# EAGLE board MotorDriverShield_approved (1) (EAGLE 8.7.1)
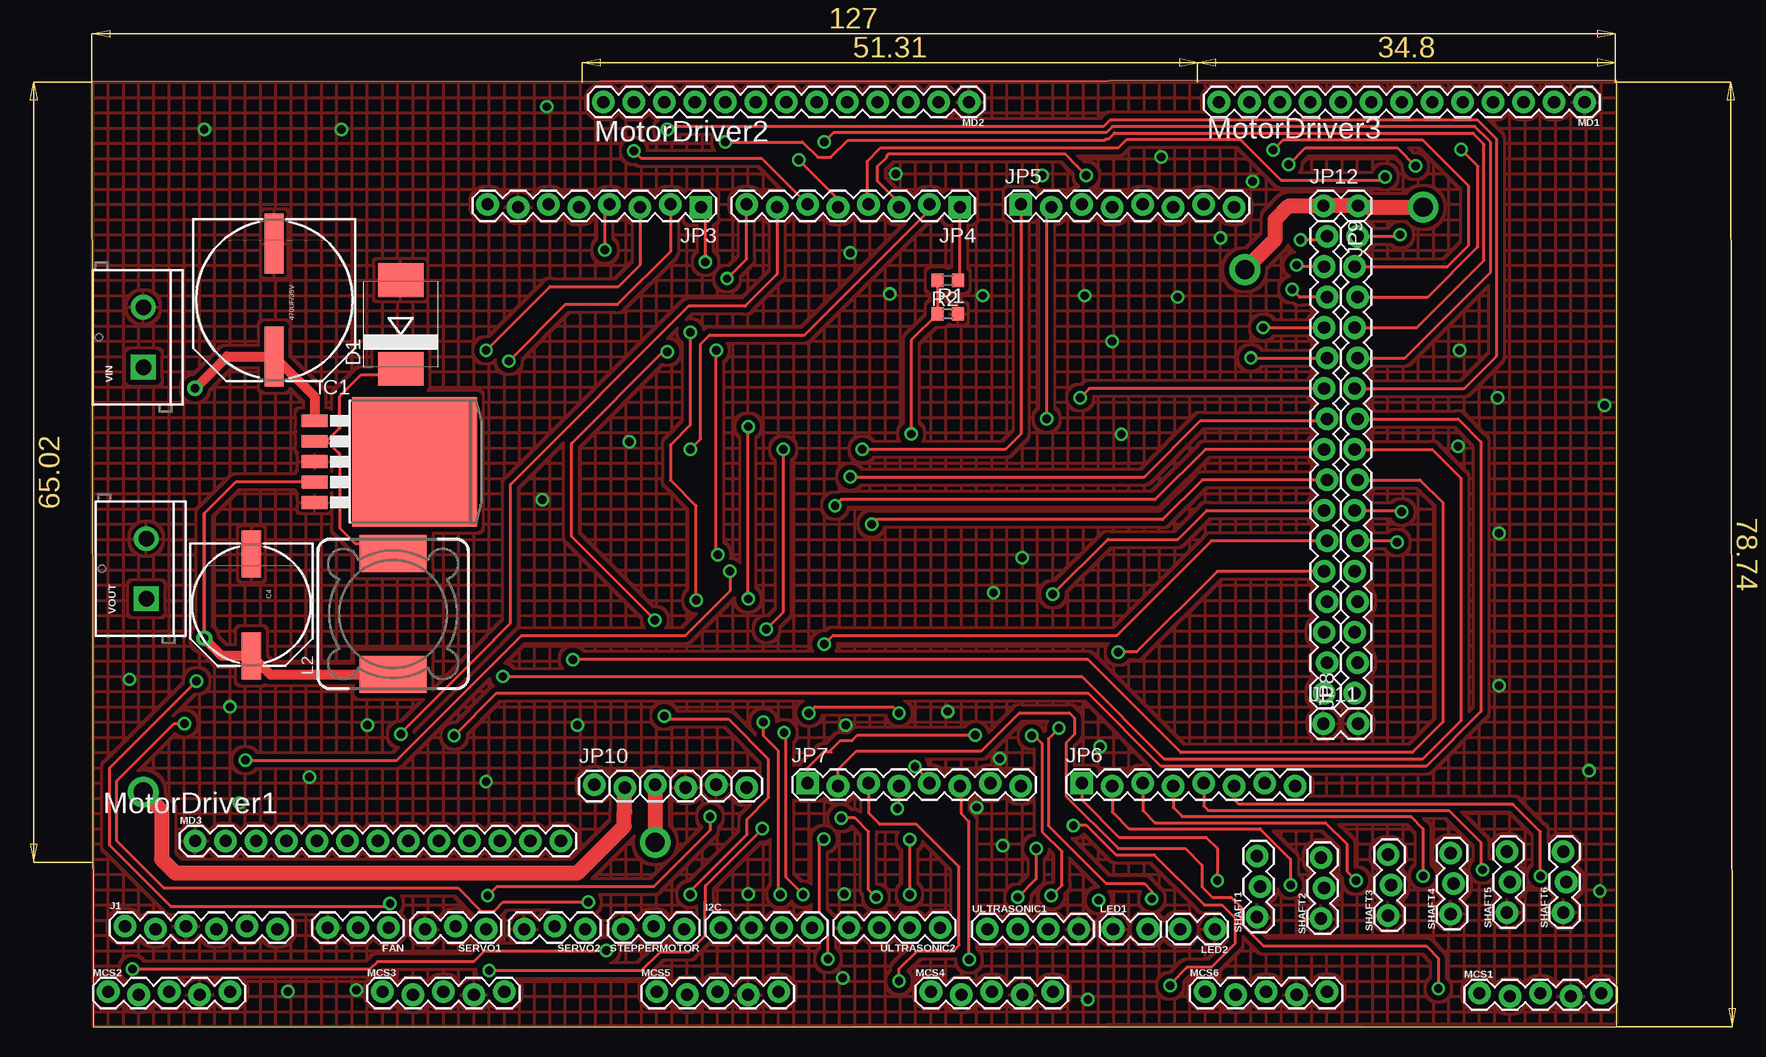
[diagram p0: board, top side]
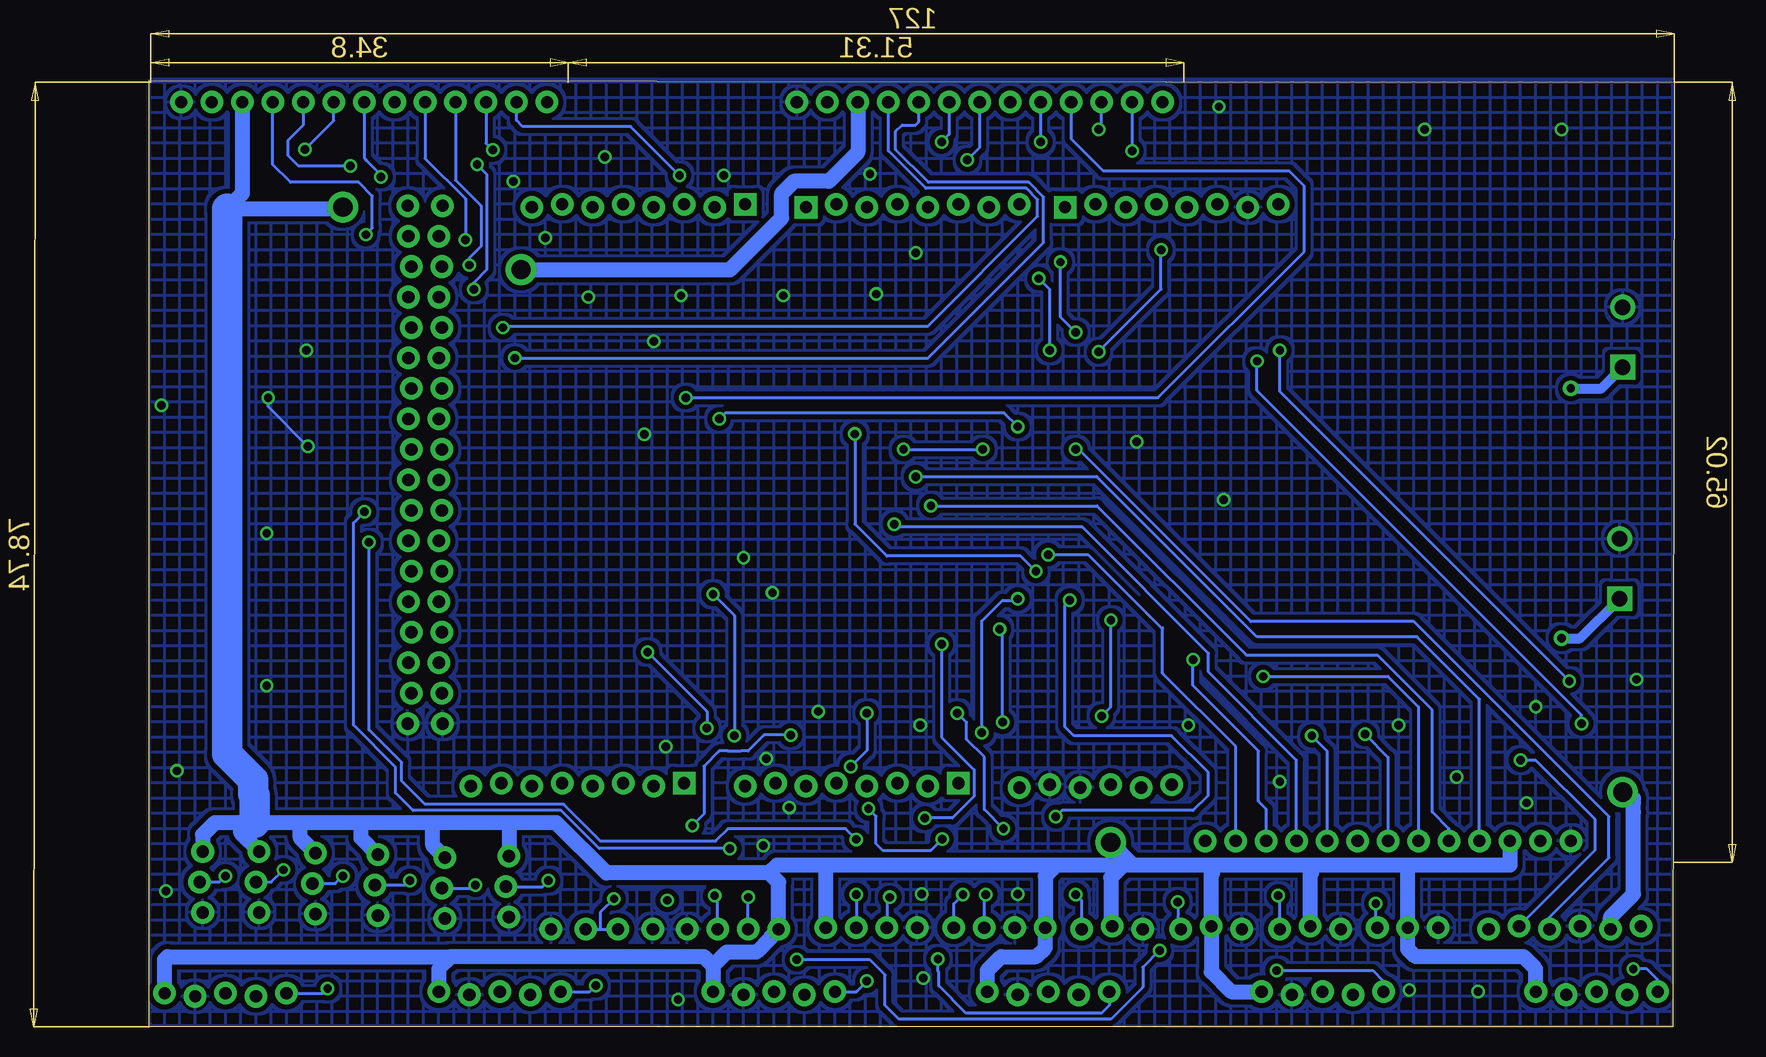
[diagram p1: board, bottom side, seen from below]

Size 142.2 x 83.1 mm. Coordinates in mm from the lower left corner, seen from the top.
Outline: 132.25,78.87 5.13,78.74 5.25,0 132.25,0 132.25,78.87
Copper layers (1*16): Top 0.035mm / dielectric 1.5mm / Bottom 0.035mm
Design rules "Voltera_DRC": minimum track width 10mil, minimum drill 0.6mm, track to track 10mil, track to pad 10mil, pad to pad 0.6mm, via to via 0.6mm, smd to smd 0mil, copper to edge 0mil, drill to drill 0.8mm, minimum pad ring 0.2mm, minimum via ring 0.2mm, stop-mask expansion 4mil, vias tented up to drill 0mil, thermal gap 10mil

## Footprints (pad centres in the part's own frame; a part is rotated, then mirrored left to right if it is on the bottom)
CPOL_PANASONIC_H13 = smd 5 x 1.6: + 4.7,0; - -4.7,0
CPOL_PANASONIC_G = smd 3.9 x 1.6: + 4.25,0; - -4.25,0
SMC = smd 2.8 x 3.8: A 3.7,0; C -3.7,0
1X03 = drill 1.016 pad 1.88: 1 0,0; 2 2.54,0; 3 5.08,0
1X04 = drill 1.016 pad 1.88: 1 0,0; 2 2.54,0; 3 5.08,0; 4 7.62,0
TO263-5 = smd 1.067 x 2.159: 1 -3.404,-5.791; 2 -1.702,-5.791; 3 0,-5.791; 4 1.702,-5.791; 5 3.404,-5.791 | smd 10.8 x 10.41: 6 0,2.54
1X06_LOCK = drill 1.016 pad 1.88: 1 0,0; 2 2.54,-0.254; 3 5.08,0; 4 7.62,-0.254; 5 10.16,0; 6 12.7,-0.254
1X08_LOCK = drill 1.016 pad 1.88 square: 1 0,0.127 | drill 1.016 pad 1.88: 2 2.54,-0.127; 3 5.08,0.127; 4 7.62,-0.127; 5 10.16,0.127; 6 12.7,-0.127; 7 15.24,0.127; 8 17.78,-0.127
1X16_LOCK = drill 1.016 pad 1.88: 1 0,0.127; 2 2.54,-0.127; 3 5.08,0.127; 4 7.62,-0.127; 5 10.16,0.127; 6 12.7,-0.127; 7 15.24,0.127; 8 17.78,-0.127; 9 20.32,0.127; 10 22.86,-0.127; 11 25.4,0.127; 12 27.94,-0.127; 13 30.48,0.127; 14 33.02,-0.127; 15 35.56,0.127; 16 38.1,-0.127
1X02_LOCK = drill 1.016 pad 1.88: 1 -0.178,0; 2 2.718,0
SRR1210 = smd 5.6 x 3.1: 1 0,5.05; 2 0,-5.05
1X05_LOCK = drill 1.016 pad 1.88: 1 0,0.127; 2 2.54,-0.127; 3 5.08,0.127; 4 7.62,-0.127; 5 10.16,0.127
1X13 = drill 1.016 pad 1.88: 1 0,0; 2 2.54,0; 3 5.08,0; 4 7.62,0; 5 10.16,0; 6 12.7,0; 7 15.24,0; 8 17.78,0; 9 20.32,0; 10 22.86,0; 11 25.4,0; 12 27.94,0; 13 30.48,0
R0603 = smd 1 x 1.1: 1 -0.85,0; 2 0.85,0
1X03_LOCK = drill 1.016 pad 1.88: 1 0,0.127; 2 2.54,-0.127; 3 5.08,0.127
SCREWTERMINAL-5MM-2 = drill 1.3 pad 2.032 square: 1 0,0 | drill 1.3 pad 2.032: 2 5,0

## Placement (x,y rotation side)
470UF/35V  [CPOL_PANASONIC_H13]  20.37,60.58 270 top
C4  220uf/25v  [CPOL_PANASONIC_G]  18.46,35.18 270 top
D1  [SMC]  30.91,58.55 90 top
FAN  [1X03]  29.89,8.26 180 top
I2C  [1X04]  57.58,8.26 0 top
IC1  LM2596S  [TO263-5]  29.51,47.12 270 top
J1  [1X06_LOCK]  7.92,8.38 0 top
JP3  [1X08_LOCK]  55.93,68.45 180 top
JP4  [1X08_LOCK]  77.52,68.45 180 top
JP5  [1X08_LOCK]  82.6,68.45 0 top
JP6  [1X08_LOCK]  87.68,20.19 0 top
JP7  [1X08_LOCK]  64.82,20.19 0 top
JP8  M16LOCK  [1X16_LOCK]  110.54,27.81 90 top
JP9  M16LOCK  [1X16_LOCK]  108,65.91 270 top
JP10  [1X06_LOCK]  47.04,20.19 0 top
JP11  [1X02_LOCK]  108,25.27 0 top
JP12  [1X02_LOCK]  108,68.45 0 top
L2  SRR1210  [SRR1210]  30.27,34.42 0 top
LED1  [1X02_LOCK]  90.47,8.13 0 top
LED2  [1X02_LOCK]  98.6,8.13 180 top
MCS1  [1X05_LOCK]  120.82,2.67 0 top
MCS2  [1X05_LOCK]  6.52,2.79 0 top
MCS3  [1X05_LOCK]  29.38,2.79 0 top
MCS4  [1X05_LOCK]  75.1,2.79 0 top
MCS5  [1X05_LOCK]  52.24,2.79 0 top
MCS6  [1X05_LOCK]  97.96,2.79 0 top
MD1  [1X13]  129.59,77.09 180 top
MD2  [1X13]  78.28,77.09 180 top
MD3  [1X13]  13.76,15.49 0 top
R1  1k  [R0603]  76.5,59.44 0 top
R2  2k  [R0603]  76.5,62.23 180 top
SERVO1  [1X03_LOCK]  38.02,8.26 180 top
SERVO2  [1X03_LOCK]  46.27,8.26 180 top
SHAFT1  [1X03_LOCK]  102.41,9.14 90 top
SHAFT2  [1X03_LOCK]  107.74,9.02 90 top
SHAFT3  [1X03_LOCK]  113.33,9.27 90 top
SHAFT4  [1X03_LOCK]  118.54,9.4 90 top
SHAFT5  [1X03_LOCK]  123.24,9.53 90 top
SHAFT6  [1X03_LOCK]  127.94,9.53 90 top
STEPPERMOTOR  [1X03_LOCK]  54.53,8.26 180 top
ULTRASONIC1  [1X04]  79.8,8.13 0 top
ULTRASONIC2  [1X04]  75.86,8.26 180 top
VIN  [SCREWTERMINAL-5MM-2]  9.44,54.99 90 top
VOUT  [SCREWTERMINAL-5MM-2]  9.7,35.69 90 top

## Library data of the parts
470UF/35V C4 = ELL-i-Passive
D1 = diode
FAN J1 LED1 LED2 MCS1-MCS6 MD1-MD3 SERVO1 SERVO2 SHAFT1-SHAFT6 STEPPERMOTOR = SparkFun-Connectors
I2C ULTRASONIC1 ULTRASONIC2 = SparkFun-Connectors; PROD_ID: CONN-09696
IC1 = national-semiconductor; MF: NATIONAL SEMICONDUCTOR; MPN: LM2596S-ADJ/NOPB; OC_FARNELL: 9494367; OC_NEWARK: 41K3842
JP3-JP12 = SparkFun
L2 = inductor-bourns
R1 R2 = audio amplifier example
VIN VOUT = SparkFun-Connectors; SF_SKU: PRT-08432

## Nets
3.3: J1.2 JP10.2
5V: FAN.2 I2C.1 JP10.3 JP12.1 JP12.2 MCS1.5 MCS2.5 MCS3.5 MCS4.5 MCS5.5 MCS6.5 MD1.3 MD2.3 MD3.3 SERVO1.2 SERVO2.2 SHAFT1.3 SHAFT2.3 SHAFT3.3 SHAFT4.3 SHAFT5.3 SHAFT6.3 STEPPERMOTOR.2 ULTRASONIC1.1 ULTRASONIC2.1
A0: JP7.1 MCS6.1
A1: JP7.2 MCS1.1
A2: JP7.3 MCS4.1
A3: JP7.4 MCS5.1
A4: JP7.5 MCS3.1
A5: JP7.6 MCS2.1
A6: JP7.7
A7: JP7.8
A8: JP6.1 SHAFT1.2
A9: JP6.2 SHAFT2.2
A10: JP6.3 SHAFT3.2
A11: JP6.4 SHAFT4.2
A12: JP6.5 SHAFT5.2
A13: JP6.6 SHAFT6.2
A14: JP6.7
A15: JP6.8
AREF: JP3.8
D2: JP4.3 MD1.12
D3: JP4.4 MD1.7
D4: JP4.5 MD2.7
D5: JP4.6 MD2.12
D6: JP4.7 MD3.7
D7: JP4.8 MD3.12
D8: JP3.1 SERVO1.1
D9: JP3.2 SERVO2.1
D10: FAN.1 JP3.3
D11: JP3.4 STEPPERMOTOR.1
D12: JP3.5
D13: JP3.6
D14: JP5.8
D15: JP5.7
D16: JP5.6
D17: JP5.5
D18: JP5.4
D19: JP5.3
D22: JP9.1 MD1.9
D23: JP8.16 MD1.4
D24: JP9.2 MD1.10
D25: JP8.15 MD1.11
D26: JP9.3 MD1.5
D27: JP8.14 MD1.6
D28: JP9.4 MD2.4
D29: JP8.13 MD2.9
D30: JP9.5 MD2.5
D31: JP8.12 MD2.6
D32: JP9.6 MD2.10
D33: JP8.11 MD2.11
D34: JP9.7 MD3.4
D35: JP8.10 MD3.9
D36: JP9.8 MD3.5
D37: JP8.9 MD3.6
D38: JP9.9 MD3.10
D39: JP8.8 MD3.11
D40: JP9.10 ULTRASONIC1.3
D41: JP8.7 ULTRASONIC1.2
D42: JP9.11 ULTRASONIC2.3
D43: JP8.6 ULTRASONIC2.2
D44: JP9.12 LED1.2 LED2.2
D45: JP8.5
D46: JP9.13
D47: JP8.4
D48: JP9.14
D49: JP8.3
D50: JP9.15
D51: JP8.2
D52: JP9.16
D53: JP8.1
EN: J1.1
GND: 470UF/35V.- C4.- D1.A FAN.3 I2C.2 IC1.3 IC1.5 J1.3 JP3.7 JP10.4 JP10.5 JP11.1 JP11.2 LED1.1 LED2.1 MCS1.4 MCS2.4 MCS3.4 MCS4.4 MCS5.4 MCS6.4 MD1.1 MD2.1 MD3.1 R1.2 SERVO1.3 SERVO2.3 SHAFT1.1 SHAFT2.1 SHAFT3.1 SHAFT4.1 SHAFT5.1 SHAFT6.1 STEPPERMOTOR.3 ULTRASONIC1.4 ULTRASONIC2.4 VIN.2 VOUT.2
OUT: D1.C IC1.2 L2.1
PVIN: 470UF/35V.+ IC1.1 VIN.1
PVOUT: C4.+ IC1.4 L2.2 VOUT.1
RES: JP10.1
RX: JP4.1 R2.1
RX0: J1.5 R1.1 R2.2
SCL: I2C.3 JP5.1
SDA: I2C.4 JP5.2
STATE: J1.6
TX: J1.4 JP4.2
VIN: JP10.6

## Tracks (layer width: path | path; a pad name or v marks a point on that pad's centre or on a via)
3.3  (via drill 1.6)
  Top 1.27: JP10.2 49.58,17.95 49.53,17.91 49.53,16.72 45.64,12.83 12.11,12.83 10.97,13.97 10.97,18.03 v9.44,19.56
  Bottom 1.27: J1.2 10.46,9.14 8.55,11.05 8.55,17.91 8.55,18.67 | 8.55,18.67 8.55,19.05 | 8.55,18.67 v9.44,19.56
5V  (via drill 1.6)
  Top 1.27: v101.27,63.12 103.81,65.66 103.81,67.31 104.95,68.45 JP12.1 JP12.2 110.84,68.33 v116.12,68.33 | JP10.3 v52.12,15.37
  Bottom 1.27: 102.03,17.02 98.34,17.02 94.15,12.83 80.58,12.83 | 102.03,17.02 108.63,17.02 | 108.63,17.02 114.6,17.02 | 114.6,17.02 119.68,17.02 | 119.68,17.02 123.49,17.02 124.63,17.02 | SHAFT2.3 108.63,15.11 108.63,17.02 | SHAFT3.3 114.6,15.75 114.6,17.02 | SHAFT4.3 119.68,15.75 119.68,17.02 | SHAFT5.3 124.63,16.13 124.63,17.02 | MD1.3 124.51,69.47 125.78,68.2 116.25,68.2 v116.12,68.33 | SERVO1.2 35.48,12.7 | 35.48,12.7 35.35,12.83 | 43.73,12.7 SERVO2.2 43.73,4.57 42.08,2.92 MCS3.5 | 43.73,12.7 43.61,12.83 | 102.03,17.02 102.28,16.76 SHAFT1.3 | 124.63,17.02 126.79,17.02 127.81,16 SHAFT6.3 | MD3.3 18.84,13.46 27.48,13.46 | MD2.3 73.2,72.9 75.61,70.48 78.53,70.48 79.55,69.47 79.55,67.44 83.87,63.12 v101.27,63.12 | 27.48,13.46 35.35,13.46 | 35.35,13.46 43.99,13.46 | 27.48,13.46 27.35,13.34 FAN.2 27.35,6.48 26.72,5.84 17.7,5.84 16.68,4.83 MCS2.5 16.68,3.43 | 35.48,12.7 35.48,13.34 35.35,13.46 | 43.73,12.7 43.73,13.21 43.99,13.46 | 50.21,13.46 v52.12,15.37 | 43.99,13.46 50.21,13.46 | 50.21,13.46 51.1,13.46 | 51.1,13.46 52.12,12.45 52.12,8.51 STEPPERMOTOR.2 | 51.1,13.46 56.69,13.46 | 56.69,13.46 57.58,12.57 I2C.1 57.58,6.6 58.34,5.84 61.26,5.84 62.4,4.7 MCS5.5 | 56.69,13.46 75.74,13.46 | 75.74,13.46 79.95,13.46 80.58,12.83 | 75.74,13.46 75.86,13.34 ULTRASONIC2.1 | 80.58,12.83 79.8,12.05 ULTRASONIC1.1 80.51,7.42 80.51,7.37 81.66,6.22 84.12,6.22 85.26,5.08 | 85.26,5.08 MCS4.5 | 85.26,5.08 86.03,5.84 107.11,5.84 | MCS6.5 108.12,4.83 107.11,5.84 | MCS1.5 130.98,5.59 130.73,5.84 107.11,5.84
  Bottom 2.54: 123.49,17.02 123.49,19.3 123.62,19.43 123.62,20.57 125.78,22.73 125.78,68.2
A0  (via drill 0.7)
  Top 0.254: JP7.1 64.82,21.59 66.13,22.91 66.59,22.91 | v86.98,16.78 88.08,16.78 90.51,14.35 93.69,14.35 97.88,10.16 99.36,10.16 100.45,9.07 100.45,6.93 98.47,4.95 96.44,4.95 95.04,3.56 v95.04,3.43 | 66.8,22.91 66.59,22.91 | 66.59,22.91 67.55,23.86 68.52,23.86 68.98,24.32 v78.8,24.32
  Bottom 0.254: v78.8,24.32 81.01,24.32 82.34,22.99 82.94,22.99 82.95,22.97 84.02,22.97 84.03,22.99 84.75,22.99 86.03,21.72 86.03,17.73 v86.98,16.78 | MCS6.1 95.55,2.92 v95.04,3.43
A1  (via drill 0.7)
  Top 0.254: JP7.2 67.36,21.46 68.88,22.99 79.29,22.99 82.49,26.18 86.64,26.18 87.06,25.76 87.06,24.36 86.36,23.66 86.36,19.22 90.72,14.86 96.31,14.86 97.69,13.48 97.69,11.66 98.56,10.79 100.12,10.79 100.96,9.96 100.96,8.6 102.83,6.73 116.38,6.73 117.39,5.71 v117.39,3.17
  Bottom 0.254: MCS1.1 117.78,2.79 v117.39,3.17
A2  (via drill 0.7)
  Top 0.254: JP7.3 69.9,17.82 70.81,16.91 73.86,16.91 77.45,13.31 77.45,6.79 77.01,6.35 73.96,6.35 72.44,4.83 v72.44,3.81
  Bottom 0.254: MCS4.1 73.33,2.92 v72.44,3.81
A3  (via drill 0.7)
  Top 0.254: v66.52,5.64 66.52,8.8 65.83,9.49 65.83,15.29 v66.18,15.64 | v72.31,18.2 72.44,18.32 JP7.4
  Bottom 0.254: v72.31,18.2 71.67,17.56 71.67,15.24 71.15,14.71 67.1,14.71 v66.18,15.64 | MCS5.1 52.24,1.78 52.88,1.14 64.18,1.14 66.45,3.41 66.45,4.6 66.52,4.67 v66.52,5.64
A4  (via drill 0.7)
  Top 0.254: v61.06,16.51 56.31,11.76 56.31,11.58 56.32,11.56 56.32,10.5 56.26,10.43 56.26,7.71 56.31,7.66 56.31,7.62 54.91,6.22 52.52,6.22 51,4.7 v38.27,4.7 | v64.93,26.16 65.43,26.67 71.93,26.67 v72.44,26.16 | v73.77,21.7 74.98,20.5 JP7.5
  Bottom 0.254: v61.06,16.51 62.66,18.11 62.66,22.5 64.14,23.98 64.14,25.38 v64.93,26.16 | v72.44,26.16 72.44,23.04 v73.77,21.7 | MCS3.1 29.38,3.81 30.27,4.7 v38.27,4.7
A5  (via drill 0.7)
  Top 0.254: v78.28,5.59 78.28,17.1 77.63,17.75 77.63,19.96 JP7.6 | v8.55,4.83 28.37,4.83 28.96,5.42 36.96,5.42 37.89,6.35 47.16,6.35 47.18,6.37 v48.05,6.37
  Bottom 0.254: v78.28,5.59 72.18,5.59 70.91,4.32 70.91,1.78 69.77,0.64 52.12,0.64 49.45,3.3 49.45,4.97 v48.05,6.37 | MCS2.1 6.52,3.94 7.41,4.83 v8.55,4.83
A8  (via drill 0.7)
  Top 0.254: JP6.1 87.68,18.92 90.79,15.81 98.03,15.81 98.98,14.86 v98.98,12.19
  Bottom 0.254: SHAFT1.2 99.49,11.68 v98.98,12.19
A9  (via drill 0.7)
  Top 0.254: JP6.2 90.22,17.91 91.61,16.51 102.53,16.51 105.08,13.97 v105.08,11.81
  Bottom 0.254: SHAFT2.2 105.33,11.56 v105.08,11.81
A10  (via drill 0.7)
  Top 0.254: JP6.3 92.76,18.03 93.77,17.02 108,17.02 109.77,15.24 109.77,12.95 v110.54,12.19
  Bottom 0.254: v110.54,12.19 110.92,11.81 SHAFT3.2
A11  (via drill 0.7)
  Top 0.254: JP6.4 95.3,18.29 96.06,17.53 115.11,17.53 116.12,16.51 v116.12,12.57
  Bottom 0.254: SHAFT4.2 116.76,11.94 v116.12,12.57
A12  (via drill 0.7)
  Top 0.254: JP6.5 97.84,18.41 98.22,18.03 118.28,18.03 120.95,15.37 120.95,13.21 v121.08,13.08
  Bottom 0.254: SHAFT5.2 122.09,12.06 v121.08,13.08
A13  (via drill 0.7)
  Top 0.254: v125.9,12.57 125.9,16.26 123.62,18.54 100.76,18.54 100.38,18.92 JP6.6
  Bottom 0.254: SHAFT6.2 126.41,12.06 v125.9,12.57
D2  (via drill 0.7)
  Top 0.254: 87.28,71.75 87.29,71.75 | 87.29,71.75 v88.06,70.98 | 87.29,71.75 87.29,71.76 86.28,72.77 75.86,72.77 75.48,72.77 71.55,72.77 71.42,72.64 71.42,72.52 70.66,71.75 70.66,70.48 72.44,68.71 JP4.3
  Bottom 0.254: MD1.12 101.65,75.56 101.14,75.06 92.14,75.06 v88.06,70.98
D3  (via drill 0.7)
  Top 0.254: JP4.4 69.77,68.71 69.77,72.14 70.91,73.28 90.72,73.28 91.44,74 100.87,74 104.27,70.59 112.68,70.59 v112.95,70.87
  Bottom 0.254: 112.95,71.03 112.95,70.99 | 112.95,70.99 v112.95,70.87 | MD1.7 114.35,72.43 114.2,72.29 114.2,72.25 112.95,70.99
D4  (via drill 0.7)
  Top 0.254: v64.07,72.28 67.36,68.99 JP4.5
  Bottom 0.254: MD2.7 63.04,73.31 v64.07,72.28
D5  (via drill 0.7)
  Top 0.254: JP4.6 61.01,72.39 50.97,72.39 v50.34,73.03
  Bottom 0.254: MD2.12 v50.34,73.03
D6  (via drill 0.7)
  Top 0.254: JP4.7 62.28,62.74 59.61,60.07 54.91,60.07 40.05,45.21 40.05,33.66 38.65,32.26 38.65,32.23 30.91,24.48 v30.91,24.38
  Bottom 0.254: v30.91,24.38 29,22.48 MD3.7
D7  (via drill 0.7)
  Top 0.254: v57.32,39.37 57.2,39.5 v57.2,56.39 | v58.11,62.38 59.74,64.01 JP4.8
  Bottom 0.254: v57.2,56.39 57.2,61.47 v58.11,62.38 | 47.8,33.15 47.8,29.46 41.7,23.37 MD3.12 | 47.8,33.15 47.8,33.27 | 47.8,33.15 54.02,39.37 v57.32,39.37
D8  (via drill 0.7)
  Top 0.254: v38.15,10.92 38.91,11.68 51.99,11.68 56.69,16.38 v56.69,17.53 | v55.53,35.56 55.53,43.43 53.39,45.58 53.39,48.51 55.04,50.16 v55.04,57.91 | v56.31,63.75 56.31,67.94 JP3.1
  Bottom 0.254: SERVO1.1 38.02,10.79 v38.15,10.92 | v55.53,35.56 55.93,35.16 55.93,25.02 55.16,24.26 47.04,24.26 43.99,21.21 43.99,19.3 45.26,18.03 56.18,18.03 v56.69,17.53 | v55.04,57.91 56.31,59.18 v56.31,63.75
D9  (via drill 0.7)
  Top 0.254: v46.53,10.4 39.44,10.4 38.68,9.63 37.61,9.63 35.67,11.57 11.16,11.57 7.24,15.49 7.24,20.49 12.03,25.27 v12.87,25.27 | v39.92,55.5 44.62,60.2 48.94,60.2 53.39,64.64 JP3.2
  Bottom 0.254: v12.87,25.27 12.87,25.99 39.92,53.04 v39.92,55.5 | v46.53,10.4 46.53,8.38 SERVO2.1
D10  (via drill 0.7)
  Top 0.254: JP3.3 50.85,63.5 49.07,61.72 43.35,61.72 v38.02,56.39 | v13.89,28.83 6.61,21.55 6.61,15.15 11.73,10.03 29.76,10.03 v30.02,10.29
  Bottom 0.254: FAN.1 30.02,8.38 v30.02,10.29 | v13.89,28.83 38.02,52.96 v38.02,56.39
D11  (via drill 0.7)
  Top 0.254: v52.1,33.91 45.13,40.88 45.13,48.64 52.77,56.28 v53.13,56.28 | v47.92,64.77 47.92,68.2 JP3.4 | v52.88,25.91 53.13,25.65 58.21,25.65 61.58,22.29 61.58,19.11 59.77,17.31 59.77,16.04 55.04,11.3 v55.04,11.03
  Bottom 0.254: STEPPERMOTOR.1 54.53,10.52 v55.04,11.03 | v52.88,25.91 52.1,26.69 v52.1,33.91 | v53.13,56.28 47.92,61.48 v47.92,64.77
D22  (via drill 0.7)
  Top 0.254: JP9.1 107.81,65.6 v105.9,65.6
  Bottom 0.254: MD1.9 109.27,72.39 105.9,69.02 v105.9,65.6
D23  (via drill 0.7)
  Top 0.254: JP8.16 114.09,65.91 v114.22,66.04
  Bottom 0.254: MD1.4 121.97,71.88 120.48,70.4 114.81,70.4 113.67,69.26 113.67,66.59 v114.22,66.04
D24  (via drill 0.7)
  Top 0.254: JP9.2 105.71,63.37 v105.58,63.5
  Bottom 0.254: MD1.10 106.73,70.57 104.61,68.45 104.61,65.06 105.58,64.09 v105.58,63.5
D25  (via drill 0.7)
  Top 0.254: JP8.15 118.16,63.37 119.93,65.15 119.93,70.09 116.11,73.91 104.43,73.91 v103.63,73.1
  Bottom 0.254: MD1.11 104.19,73.66 v103.63,73.1
D26  (via drill 0.7)
  Top 0.254: JP9.3 105.84,60.83 v105.2,61.47 | v104.93,71.88 106.33,73.28 113.97,73.28 v115.49,71.75
  Bottom 0.254: v105.2,61.47 105.2,62.06 104.11,63.16 104.11,71.06 v104.93,71.88 | MD1.5 119.43,75.18 120.7,73.91 120.7,72.64 119.81,71.75 v115.49,71.75
D27  (via drill 0.7)
  Top 0.254: JP8.14 116.5,60.83 120.7,65.02 120.7,71.74 v119.3,73.14
  Bottom 0.254: v119.3,73.14 116.89,75.55 MD1.6
D28  (via drill 0.7)
  Top 0.254: v102.79,58.29 JP9.4
  Bottom 0.254: v102.79,58.29 102.64,58.44 67.34,58.44 58.21,67.56 58.21,68.96 59.15,69.9 67.53,69.9 70.66,73.03 MD2.4
D29  (via drill 0.7)
  Top 0.254: JP8.13 115.62,58.29 121.2,63.88 121.2,73.58 120.27,74.51 90.47,74.51 90.39,74.51 89.92,74.04 89.71,74.04 89.58,73.91 68.18,73.91 66.75,72.48 65.68,72.48 64.39,73.77 v57.96,73.77
  Bottom 0.254: MD2.9 v57.96,73.77
D30  (via drill 0.7)
  Top 0.254: v101.77,55.75 JP9.5
  Bottom 0.254: v101.77,55.75 67.34,55.75 57.7,65.39 57.7,69.17 58.94,70.41 67.32,70.41 70.05,73.13 70.05,74.65 69.52,75.18 68.37,75.18 68.12,75.44 MD2.5
D31  (via drill 0.7)
  Top 0.254: v66.21,73.77 66.99,74.55 89.71,74.55 90.22,75.06 120.44,75.06 121.71,73.79 121.71,62.87 114.6,55.75 JP8.12
  Bottom 0.254: MD2.6 65.58,74.41 v66.21,73.77
D32  (via drill 0.7)
  Top 0.254: JP9.6 88.31,53.21 v87.55,52.45
  Bottom 0.254: MD2.10 55.42,74.04 52.75,71.37 37.26,71.37 35.99,70.1 35.99,64.64 48.18,52.45 v87.55,52.45
D33  (via drill 0.7)
  Top 0.254: v53.13,74.8 53.39,75.06 89.5,75.06 90.01,75.56 120.7,75.56 122.22,74.04 122.22,55.88 119.55,53.21 JP8.11
  Bottom 0.254: v53.13,74.8 52.88,75.06 MD2.11
D34  (via drill 0.7)
  Top 0.254: v68.37,45.85 92.88,45.85 97.58,50.55 107.36,50.55 107.49,50.67 JP9.7
  Bottom 0.254: MD3.4 21.38,27.3 26.59,32.51 39.92,32.51 53.26,45.85 v68.37,45.85
D35  (via drill 0.7)
  Top 0.254: JP8.10 119.05,50.67 120.95,48.77 120.95,26.29 116.38,21.72 94.28,21.72 88.18,27.81 38.91,27.81 v35.35,24.26
  Bottom 0.254: v35.35,24.26 34.08,22.99 MD3.9
D36  (via drill 0.7)
  Top 0.254: JP9.8 97.96,48.13 93.77,43.94 67.61,43.94 v67.1,43.43
  Bottom 0.254: v67.1,43.43 53.26,43.43 40.81,30.99 29.89,30.99 25.32,26.42 25.32,17.91 23.92,16.51 MD3.5
D37  (via drill 0.7)
  Top 0.254: JP8.9 116.89,48.13 119.3,45.72 119.3,25.53 116.12,22.35 94.53,22.35 87.68,29.21 v39.42,29.21
  Bottom 0.254: MD3.6 26.46,26.67 29,29.21 v39.42,29.21
D38  (via drill 0.7)
  Top 0.254: JP9.9 97.71,45.59 94.41,42.29 70.53,42.29 v70.15,41.91
  Bottom 0.254: MD3.10 36.62,22.23 43.97,29.57 43.97,31.14 54.49,41.66 69.9,41.66 v70.15,41.91
D39  (via drill 0.7)
  Top 0.254: JP8.8 115.87,45.59 117.78,43.69 117.78,25.4 115.23,22.86 95.93,22.86 88.18,30.61 v45.26,30.61
  Bottom 0.254: MD3.11 39.16,18.16 39.8,18.8 39.8,22.99 45.26,28.45 v45.26,30.61
D40  (via drill 0.7)
  Top 0.254: v85.26,36.07 89.83,40.64 95.68,40.64 98.09,43.05 JP9.10 | v83.48,24.26 83.74,24.26 84.37,23.62 84.37,16.26 86.03,14.61 86.03,11.81 v85.14,10.92
  Bottom 0.254: v85.26,36.07 83.48,34.29 v83.48,24.26 | ULTRASONIC1.3 84.88,10.67 v85.14,10.92
D41  (via drill 0.7)
  Top 0.254: 110.92,43.05 JP8.7 114.2,43.05 v114.33,42.93 | v82.34,10.79 83.87,12.32 v83.87,14.86
  Bottom 0.254: v114.33,42.93 115.23,42.02 115.23,25.15 111.73,21.64 111.73,19.48 110.28,18.03 97.92,18.03 94.75,14.86 v83.87,14.86 | ULTRASONIC1.2 v82.34,10.79
D42  (via drill 0.7)
  Top 0.254: JP9.11 98.47,40.51 90.6,32.64 66.96,32.64 v66.21,31.89 | v70.53,10.79 69.9,11.43 69.9,16.26 68.75,17.4 v67.61,17.4
  Bottom 0.254: v70.53,10.79 70.78,10.54 ULTRASONIC2.3 | v66.21,31.89 66.21,24.14 63.49,21.42 63.49,19.22 65.32,17.4 v67.61,17.4
D43  (via drill 0.7)
  Top 0.254: v73.33,15.62 v73.33,11.03 | v113.95,40.39 113.82,40.51 JP8.6
  Bottom 0.254: v73.33,11.03 ULTRASONIC2.2 | v113.95,40.39 113.95,24.75 111.22,22.02 111.22,20.5 109.27,18.54 97.71,18.54 94.67,15.49 85.05,15.49 84.03,16.51 74.21,16.51 v73.33,15.62
D44  (via drill 0.7)
  Top 0.254: JP9.12 98.98,37.97 92.25,31.24 v90.72,31.24 | v93.52,10.67 93.52,11.3 92.88,11.94 89.71,11.94 85.14,16.51 84.88,16.76 84.88,24 v85.77,24.89
  Bottom 0.254: LED2.2 94.66,8.13 | 94.66,8.13 LED1.2 | 93.64,10.54 v93.52,10.67 94.66,9.53 94.66,8.13 | v85.77,24.89 85.77,26.29 v90.72,31.24
GND  (via drill 0.7)
  Top 0.813: IC1.5 23.72,43.61
  Bottom 0.254: v119.05,48.39 122.35,51.69 v122.35,52.45
  other vias: 101.9,70.48 95.68,60.83 87.93,60.96 71.67,61.09 68.37,64.52 43.1,76.71 90.98,49.4 42.72,43.94 49.96,48.77 78.91,18.29 80.31,36.2 82.72,39.12 23.29,20.83 79.42,60.96 67.99,25.15 90.22,57.15 99.23,65.79 45.64,25.15 38.02,20.45 28.11,25.15 84.37,70.99 122.47,41.15 122.47,28.45 25.95,74.8 14.52,74.8 80.82,22.35 81.07,15.11 119.17,56.39 131.24,51.82 76.5,26.29 89.2,23.37 27.22,3.05 21.51,2.92 8.3,28.96 16.68,26.67 17.45,18.67 59.86,11.05 67.74,4.06 67.86,11.05 88.18,2.29 130.86,11.3 129.97,21.34 94.28,72.52 72.18,71.12
  pour Top (isolate 0.406, hatched): 5.25,0 132.25,0.25 132.25,78.87 5.13,78.74
  pour Bottom (isolate 0.406, hatched): 5.25,0 5.25,78.99 131.87,78.99 132.25,78.87 132.25,0.13
N$5  (via drill 0.7)
  other vias: 89.07,10.54
OUT
  Top 0.254: 27.12,40.28 25.8,41.6 25.8,47.67 arc45 25.73,47.85 24.84,48.74 arc45 24.66,48.82 IC1.2 24.73,48.82 25.83,49.91 25.83,52.58 27.61,54.36 30.42,54.36 D1.C | 27.12,40.28 27.15,40.26 | 27.12,40.28 28.62,40.28 28.82,40.28 29.46,40.28 L2.1
PVIN  (via drill 0.7 pad 1.3)
  Top 0.813: 24.02,50.52 IC1.1 23.72,52.53 470UF/35V.+ 16.43,55.88 v13.76,53.21
  Bottom 0.813: v13.76,53.21 11.22,53.21 VIN.1
PVOUT  (via drill 0.7 pad 1.3)
  Top 0.254: IC1.4 17.14,45.41 14.52,42.8
  Top 0.305: v14.52,32.38 14.52,42.8
  Top 0.813: v14.53,32.39 v14.52,32.38 15.98,30.93 C4.+ 20.02,29.37 L2.2
  Bottom 0.813: v14.52,32.38 13,32.38 VOUT.1
RX
  Top 0.254: R2.1 77.52,62.4 JP4.1
RX0  (via drill 0.7)
  Top 0.254: R2.2 R1.1 73.45,57.24 v73.45,49.42 | v17.95,22.23 30.57,22.23 40.97,32.62 52.63,32.62 52.65,32.64 54.66,32.64 58.35,36.33 v58.35,37.96
  Bottom 0.254: J1.5 11.73,14.73 11.73,17.27 16.68,22.23 v17.95,22.23 | v58.35,37.96 59.63,39.24 70.78,39.24 73.45,41.91 v73.45,49.42
SCL  (via drill 0.7)
  Top 0.254: JP5.1 82.6,49.4 81.33,48.13 v69.39,48.13 | v62.78,48.13 62.78,34.54 v61.39,33.15 | v61.13,25.4 61.13,24.26 62.34,23.05 62.34,11.22 v62.53,11.03
  Bottom 0.254: I2C.3 62.66,10.9 v62.53,11.03 | v69.39,48.13 v62.78,48.13 | v61.13,25.4 61.13,32.89 v61.39,33.15
SDA  (via drill 0.7)
  Top 0.254: v59.86,35.67 v59.86,50.04 | v84.75,50.67 84.75,67.94 JP5.2 | v64.44,11.03 63.03,12.44 63.03,24.33 v62.85,24.51
  Bottom 0.254: I2C.4 65.2,10.27 v64.44,11.03 | v62.85,24.51 62.85,33.84 61.13,35.56 59.97,35.56 v59.86,35.67 | v59.86,50.04 61.01,51.18 84.25,51.18 v84.75,50.67
TX  (via drill 0.7)
  Top 0.254: v55.04,48.13 55.91,49.01 55.91,56.92 56.66,57.67 64.58,57.67 74.98,68.07 JP4.2
  Bottom 0.254: J1.4 15.54,9.14 10.59,14.1 10.59,17.53 26.84,33.78 40.43,33.78 54.78,48.13 v55.04,48.13

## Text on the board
tPlace: MotorDriver2 | MotorDriver3 | MotorDriver1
